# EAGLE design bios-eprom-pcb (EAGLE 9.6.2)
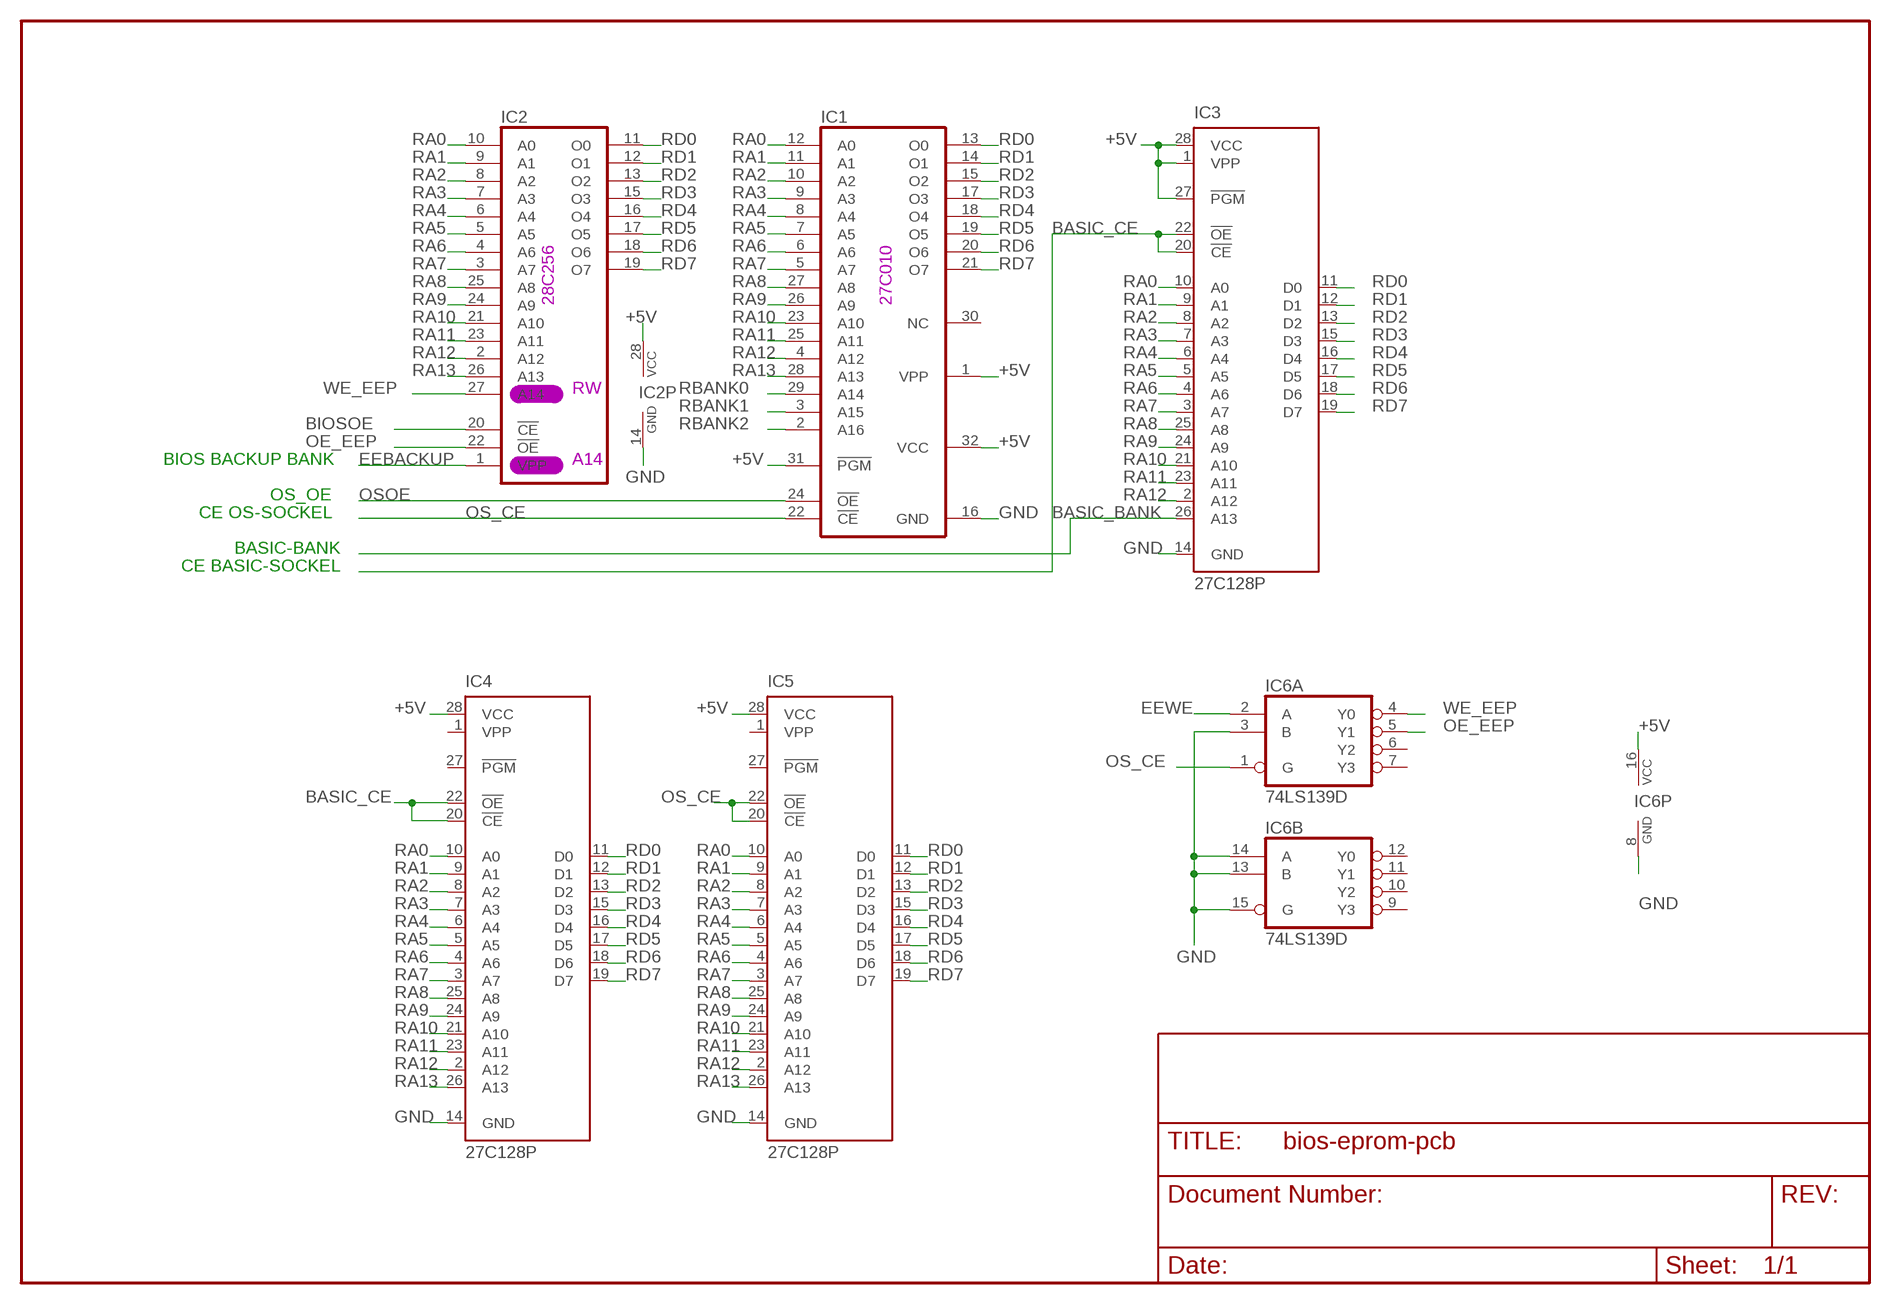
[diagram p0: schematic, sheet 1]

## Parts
IC1  27C1001A  [DIL32]
IC2  27256  [DIL28]
IC3  27C128P  [DIL28-6]
IC4  27C128P  [DIL28-6]
IC5  27C128P  [DIL28-6]
IC6  74LS139D  [SO16]

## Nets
+5V: IC1.1(VPP) IC1.31(!PGM) IC1.32(VCC) IC2.28(VCC) IC3.1(VPP) IC3.27(!PGM) IC3.28(VCC) IC4.28(VCC) IC5.28(VCC) IC6.16(P:VCC)
BASIC_BANK: IC3.26(A13)
BASIC_CE: IC3.20(!CE) IC3.22(!OE) IC4.20(!CE) IC4.22(!OE)
BIOSOE: IC2.20(!CE)
EEBACKUP: IC2.1(VPP)
EEWE: IC6.2(A:A)
GND: IC1.16(GND) IC2.14(GND) IC3.14(GND) IC4.14(GND) IC5.14(GND) IC6.3(A:B) IC6.8(P:GND) IC6.13(B:B) IC6.14(B:A) IC6.15(B:G)
OE_EEP: IC2.22(!OE) IC6.5(A:Y1)
OS_CE: IC1.22(!CE) IC5.20(!CE) IC5.22(!OE) IC6.1(A:G)
OSOE: IC1.24(!OE)
RA0: IC1.12(A0) IC2.10(A0) IC3.10(A0) IC4.10(A0) IC5.10(A0)
RA1: IC1.11(A1) IC2.9(A1) IC3.9(A1) IC4.9(A1) IC5.9(A1)
RA2: IC1.10(A2) IC2.8(A2) IC3.8(A2) IC4.8(A2) IC5.8(A2)
RA3: IC1.9(A3) IC2.7(A3) IC3.7(A3) IC4.7(A3) IC5.7(A3)
RA4: IC1.8(A4) IC2.6(A4) IC3.6(A4) IC4.6(A4) IC5.6(A4)
RA5: IC1.7(A5) IC2.5(A5) IC3.5(A5) IC4.5(A5) IC5.5(A5)
RA6: IC1.6(A6) IC2.4(A6) IC3.4(A6) IC4.4(A6) IC5.4(A6)
RA7: IC1.5(A7) IC2.3(A7) IC3.3(A7) IC4.3(A7) IC5.3(A7)
RA8: IC1.27(A8) IC2.25(A8) IC3.25(A8) IC4.25(A8) IC5.25(A8)
RA9: IC1.26(A9) IC2.24(A9) IC3.24(A9) IC4.24(A9) IC5.24(A9)
RA10: IC1.23(A10) IC2.21(A10) IC3.21(A10) IC4.21(A10) IC5.21(A10)
RA11: IC1.25(A11) IC2.23(A11) IC3.23(A11) IC4.23(A11) IC5.23(A11)
RA12: IC1.4(A12) IC2.2(A12) IC3.2(A12) IC4.2(A12) IC5.2(A12)
RA13: IC1.28(A13) IC2.26(A13) IC4.26(A13) IC5.26(A13)
RBANK0: IC1.29(A14)
RBANK1: IC1.3(A15)
RBANK2: IC1.2(A16)
RD0: IC1.13(O0) IC2.11(O0) IC3.11(D0) IC4.11(D0) IC5.11(D0)
RD1: IC1.14(O1) IC2.12(O1) IC3.12(D1) IC4.12(D1) IC5.12(D1)
RD2: IC1.15(O2) IC2.13(O2) IC3.13(D2) IC4.13(D2) IC5.13(D2)
RD3: IC1.17(O3) IC2.15(O3) IC3.15(D3) IC4.15(D3) IC5.15(D3)
RD4: IC1.18(O4) IC2.16(O4) IC3.16(D4) IC4.16(D4) IC5.16(D4)
RD5: IC1.19(O5) IC2.17(O5) IC3.17(D5) IC4.17(D5) IC5.17(D5)
RD6: IC1.20(O6) IC2.18(O6) IC3.18(D6) IC4.18(D6) IC5.18(D6)
RD7: IC1.21(O7) IC2.19(O7) IC3.19(D7) IC4.19(D7) IC5.19(D7)
WE_EEP: IC2.27(A14) IC6.4(A:Y0)
Unconnected: IC1.30(NC) IC4.1(VPP) IC4.27(!PGM) IC5.1(VPP) IC5.27(!PGM) IC6.6(A:Y2) IC6.7(A:Y3) IC6.9(B:Y3) IC6.10(B:Y2) IC6.11(B:Y1) IC6.12(B:Y0)

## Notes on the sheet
- 28C256 | 27C010
- RW
- BIOS BACKUP BANK | A14
- OS_OE
- CE OS-SOCKEL
- BASIC-BANK
- CE BASIC-SOCKEL

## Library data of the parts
IC1 = memory-nec:27C1001A: MEMORY; MPN: M27C1001-15F1; OC_FARNELL: 1661756; OC_NEWARK: 78M7615
IC2 = memory:27256: MEMORY
IC3-IC5 = microchip:27*128: CMOS EPROM 128 K (16 K x 8); OC_FARNELL: unknown; OC_NEWARK: unknown
IC6 = 74xx-eu:74*139: Dual 2-line to 4-line DECODER/DEMULTIPLEXER

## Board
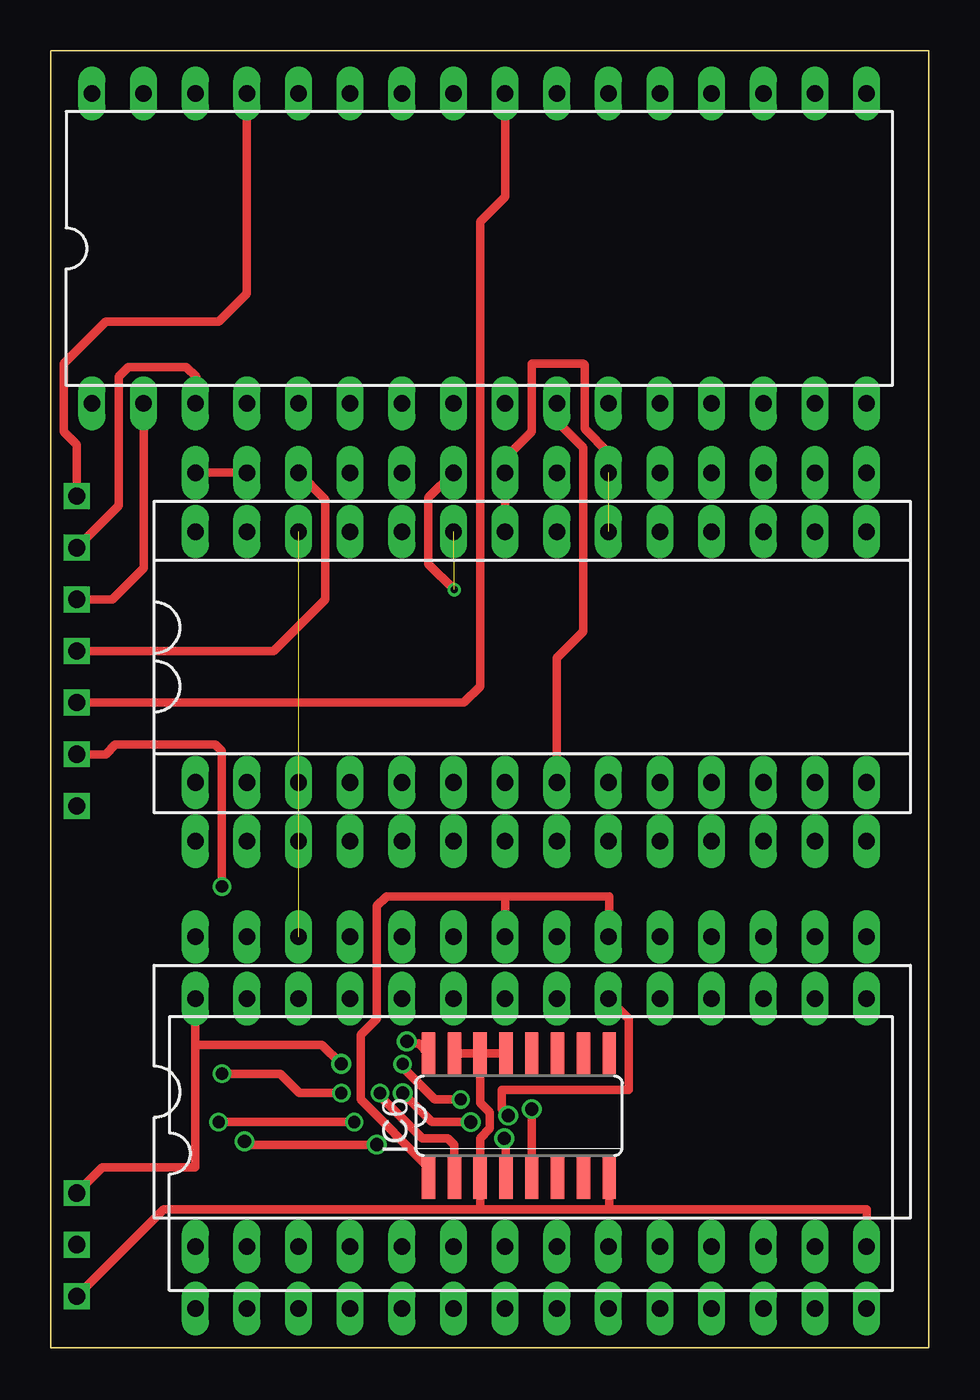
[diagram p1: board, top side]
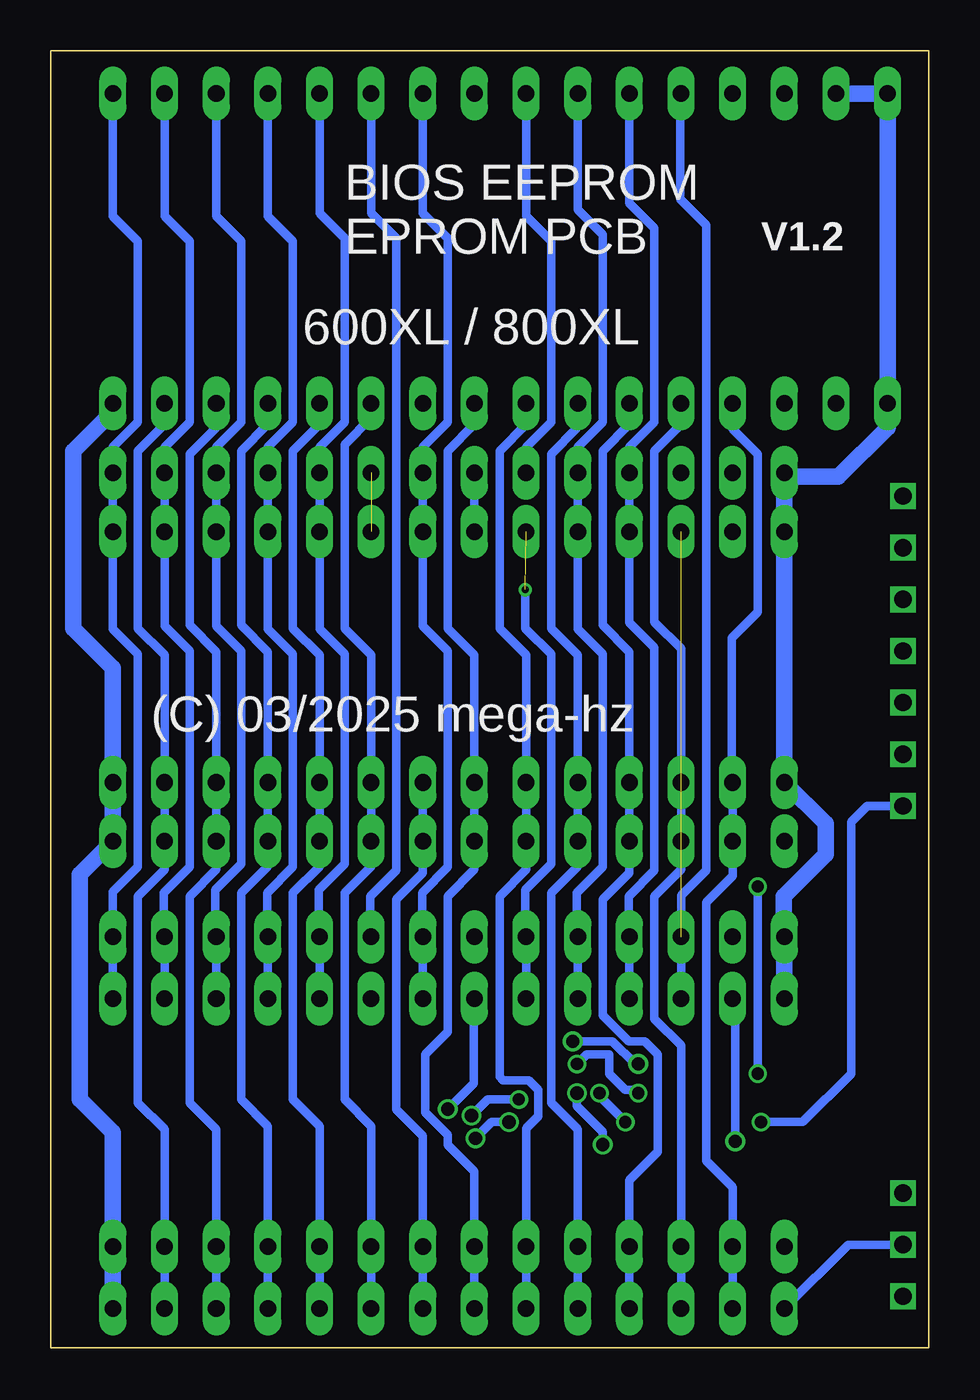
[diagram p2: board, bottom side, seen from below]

Size 43.18 x 63.82 mm. Coordinates in mm from the lower left corner, seen from the top.
Outline: 43.18,0 43.18,63.82 0,63.82 0,0 43.18,0
Copper layers (1+2*15+16): Top 0.035mm / dielectric 1.5mm / Route2 0.035mm / dielectric 0.15mm / Route15 0.035mm / dielectric 0.2mm / Bottom 0.035mm
Design rules "ITead_rule *": minimum track width 6mil, minimum drill 12mil, track to track 6mil, track to pad 6mil, pad to pad 6mil, via to via 6mil, smd to smd 0mil, copper to edge 10mil, drill to drill 10mil, minimum pad ring 10mil, minimum via ring 6mil, stop-mask expansion 2mil, vias tented up to drill 100mil, thermal gap 10mil

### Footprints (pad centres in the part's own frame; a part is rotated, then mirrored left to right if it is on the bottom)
DIL32 = drill 0.813 long: 1 -19.05,-7.62; 2 -16.51,-7.62; 3 -13.97,-7.62; 4 -11.43,-7.62; 5 -8.89,-7.62; 6 -6.35,-7.62; 7 -3.81,-7.62; 8 -1.27,-7.62; 9 1.27,-7.62; 10 3.81,-7.62; 11 6.35,-7.62; 12 8.89,-7.62; 13 11.43,-7.62; 14 13.97,-7.62; 15 16.51,-7.62; 16 19.05,-7.62; 17 19.05,7.62; 18 16.51,7.62; 19 13.97,7.62; 20 11.43,7.62; 21 8.89,7.62; 22 6.35,7.62; 23 3.81,7.62; 24 1.27,7.62; 25 -1.27,7.62; 26 -3.81,7.62; 27 -6.35,7.62; 28 -8.89,7.62; 29 -11.43,7.62; 30 -13.97,7.62; 31 -16.51,7.62; 32 -19.05,7.62
DIL28 = drill 0.813 long: 1 -16.51,-7.62; 2 -13.97,-7.62; 3 -11.43,-7.62; 4 -8.89,-7.62; 5 -6.35,-7.62; 6 -3.81,-7.62; 7 -1.27,-7.62; 8 1.27,-7.62; 9 3.81,-7.62; 10 6.35,-7.62; 11 8.89,-7.62; 12 11.43,-7.62; 13 13.97,-7.62; 14 16.51,-7.62; 15 16.51,7.62; 16 13.97,7.62; 17 11.43,7.62; 18 8.89,7.62; 19 6.35,7.62; 20 3.81,7.62; 21 1.27,7.62; 22 -1.27,7.62; 23 -3.81,7.62; 24 -6.35,7.62; 25 -8.89,7.62; 26 -11.43,7.62; 27 -13.97,7.62; 28 -16.51,7.62
DIL28-6 = drill 0.813 long: 1 -16.51,-7.62; 2 -13.97,-7.62; 3 -11.43,-7.62; 4 -8.89,-7.62; 5 -6.35,-7.62; 6 -3.81,-7.62; 7 -1.27,-7.62; 8 1.27,-7.62; 9 3.81,-7.62; 10 6.35,-7.62; 11 8.89,-7.62; 12 11.43,-7.62; 13 13.97,-7.62; 14 16.51,-7.62; 15 16.51,7.62; 16 13.97,7.62; 17 11.43,7.62; 18 8.89,7.62; 19 6.35,7.62; 20 3.81,7.62; 21 1.27,7.62; 22 -1.27,7.62; 23 -3.81,7.62; 24 -6.35,7.62; 25 -8.89,7.62; 26 -11.43,7.62; 27 -13.97,7.62; 28 -16.51,7.62
SO16 = smd 0.66 x 2.032: 1 -4.445,-3.073; 2 -3.175,-3.073; 3 -1.905,-3.073; 4 -0.635,-3.073; 5 0.635,-3.073; 6 1.905,-3.073; 7 3.175,-3.073; 8 4.445,-3.073; 9 4.445,3.073; 10 3.175,3.073; 11 1.905,3.073; 12 0.635,3.073; 13 -0.635,3.073; 14 -1.905,3.073; 15 -3.175,3.073; 16 -4.445,3.073

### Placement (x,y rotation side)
IC1  21.07,54.09 0 top
IC2  23.61,9.56 0 top
IC3  23.61,35.44 0 top
IC4  23.61,32.54 0 top
IC5  23.61,12.6 0 top
IC6  23.02,11.43 0 top

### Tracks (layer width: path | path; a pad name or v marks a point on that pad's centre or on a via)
+5V  (via drill 0.65, 0.85)
  Top 0.406: v1.27,7.62 2.54,8.89 7.1,8.89 7.1,14.92 | 7.1,14.92 IC2.28 | IC6.16 18.1,14.98 17.51,14.98 v17.51,15.08 | v14.29,13.97 13.34,14.92 7.1,14.92 | IC3.28 IC3.27
  Bottom 0.406: v17.51,15.08 15.56,15.08 14.45,13.97 v14.29,13.97
  Bottom 0.813: IC1.31 IC1.32 IC1.1 2.02,45.28 4.45,42.86 6.91,42.86 IC3.28 IC4.28 IC3.1 5.08,25.8 5.08,24.29 7.14,22.23 7.14,20.26 IC5.28 IC2.28
BASIC_BANK  (via drill 0.85)
  Top 0.406: v1.27,34.29 10.95,34.29 13.49,36.83 13.49,41.75 IC3.26
BASIC_CE  (1 unrouted)
  Top 0.406: IC4.22 22.34,43.77 23.65,45.09 23.65,48.42 26.19,48.42 26.25,48.36 26.25,45.23 27.42,44.06 IC3.20
  Bottom 0.406: IC4.22 IC3.22
BIOSOE  (via drill 0.6, 0.65, 0.85)
  Top 0.406: v20.16,12.22 18.89,12.22 17.3,13.81 v17.3,13.97 | v14.29,12.54 12.22,12.54 11.27,13.49 v8.41,13.49 | v8.41,22.7 8.41,29.37 8.1,29.69 3.17,29.69 2.7,29.21 v1.27,29.21 | v22.49,11.43 22.18,11.75 22.18,12.7 28.42,12.7 28.42,16.19 IC2.20
  Bottom 0.406: v20.16,12.22 21.7,12.22 v22.49,11.43 | v17.3,13.97 16.83,14.45 15.72,14.45 15.72,13.49 14.92,12.7 14.45,12.7 v14.29,12.54 | v8.41,13.49 v8.41,22.7
EEBACKUP  (via drill 0.85)
  Bottom 0.406: v1.27,5.08 3.97,5.08 IC2.1
EEWE  (via drill 0.6, 0.85)
  Top 0.406: IC6.2 19.84,10 19.53,10.32 18.26,10.32 16.19,12.38 v16.19,12.54 | v14.92,11.11 v8.26,11.11
  Bottom 0.406: v16.19,12.54 16.19,12.38 v14.92,11.11 | v8.26,11.11 6.19,11.11 3.81,13.49 3.81,25.88 3.02,26.67 v1.27,26.67
GND  (via drill 0.85)
  Top 0.406: v1.27,2.54 5.56,6.83 21.11,6.83 | IC5.14 40.12,6.83 27.46,6.83 | 21.11,6.83 27.46,6.83 | IC6.8 27.46,6.83 | 21.11,6.83 IC6.3 21.11,10.32 21.59,10.79 21.59,11.59 21.11,12.06 IC6.14 | IC6.15 IC6.14 | IC6.14 IC6.13
  Bottom 0.813: IC1.16 40.12,46.08 42.07,44.13 42.07,35.4 40.12,33.46 IC3.14 IC4.14 41.75,23.3 41.75,12.22 40.12,10.6 IC5.14 IC2.14
OE_EEP  (via drill 0.65)
  Top 0.406: v23.65,11.75 IC6.5
  Bottom 0.406: v23.65,11.75 22.38,13.02 22.38,17.14 IC2.22
OS_CE
  Top 0.406: IC6.1 18.57,8.89 15.24,12.22 15.24,15.4 16.03,16.19 16.03,21.75 16.51,22.23 22.38,22.23 | IC5.22 22.34,22.18 22.38,22.23 | 22.38,22.23 27.46,22.23 27.46,20.26 IC5.20
  Bottom 0.406: IC1.22 27.42,55.84 26.19,54.61 26.19,23.5 27.46,22.23 27.46,20.26 IC5.20
OSOE  (via drill 0.85)
  Top 0.406: IC1.24 22.34,56.63 21.11,55.4 21.11,32.54 20.32,31.75 v1.27,31.75
RA0
  Bottom 0.406: IC2.10 IC5.10 29.96,10.91 31.27,12.22 31.27,22.38 29.96,23.69 IC4.10 IC3.10 29.96,34.09 31.27,35.4 31.27,44.13 29.96,45.44 IC1.12
RA1
  Bottom 0.406: IC1.11 27.42,45.76 28.73,44.45 28.73,35.4 27.42,34.09 IC3.9 IC4.9 27.42,23.69 28.73,22.38 28.73,12.22 27.42,10.91 IC5.9 IC2.9
RA2
  Top 0.406: IC3.8 24.88,33.93 26.19,35.24 26.19,44.29 24.88,45.6 IC1.10
  Bottom 0.406: IC2.8 IC5.8 24.88,10.44 26.19,11.75 26.19,22.07 24.88,23.38 IC4.8 IC3.8
RA3
  Bottom 0.406: IC1.9 22.34,45.44 23.65,44.13 23.65,35.4 22.34,34.09 IC3.7 IC4.7 22.34,23.54 23.65,22.23 23.65,15.56 24.77,14.45 24.77,11.59 23.65,10.48 23.65,10 22.34,8.69 IC5.7 IC2.7
RA4
  Bottom 0.406: IC2.6 IC5.6 19.8,10.79 19.21,11.39 19.21,12.7 19.68,13.18 20.95,13.18 21.11,13.34 21.11,22.23 19.8,23.54 IC4.6 IC3.6 19.8,34.09 21.11,35.4 21.11,44.13 19.8,45.44 IC1.8
RA5
  Bottom 0.406: IC1.7 17.3,46.44 17.3,45.24 18.57,43.97 18.57,35.4 17.26,34.09 IC3.5 IC4.5 17.26,23.69 18.57,22.38 18.57,12.06 17.26,10.76 IC5.5 IC2.5
RA6
  Bottom 0.406: IC2.4 IC5.4 14.72,8.26 13.34,9.64 13.34,14.45 13.97,15.08 14.76,15.08 16.03,16.35 16.03,22.07 14.72,23.38 IC4.4 IC3.4 14.72,34.25 16.03,35.56 16.03,44.13 14.72,45.44 IC1.6
RA7
  Bottom 0.406: IC1.5 12.18,45.44 13.49,44.13 13.49,35.72 12.18,34.41 IC3.3 IC4.3 12.18,23.54 13.49,22.23 13.49,16.19 12.18,14.88 IC5.3 IC2.3
RA8
  Bottom 0.406: IC1.27 14.72,56.32 13.49,55.09 13.49,45.56 14.72,44.33 IC3.25 IC4.25 14.72,35.68 13.49,34.45 13.49,23.5 14.76,22.23 14.76,20.26 IC5.25 IC2.25
RA9
  Bottom 0.406: IC1.26 17.26,56 16.03,54.77 16.03,45.56 17.26,44.33 IC3.24 IC4.24 17.26,35.36 16.03,34.13 16.03,23.65 17.3,22.38 17.3,20.26 IC5.24 IC2.24
RA10
  Bottom 0.406: IC1.23 24.88,55.84 23.65,54.61 23.65,45.56 24.88,44.33 IC3.21 IC4.21 24.88,35.52 23.65,34.29 23.65,23.65 24.92,22.38 24.92,20.26 IC5.21 IC2.21
RA11  (via drill 0.35)  (1 unrouted)
  Top 0.406: v19.84,37.31 18.57,38.58 18.57,41.83 IC3.23
  Bottom 0.406: IC1.25 19.8,55.68 18.57,54.45 18.57,45.56 19.8,44.33 IC3.23 | IC2.23 IC5.23 19.84,20.26 19.84,22.54 18.57,23.81 18.57,34.13 19.84,35.4 v19.84,37.31
RA12
  Bottom 0.406: IC1.4 9.64,45.2 8.41,43.97 8.41,36.2 9.68,34.92 9.68,27.86 IC3.2 IC4.2 9.64,23.22 10.95,21.91 10.95,9.21 9.64,7.9 IC5.2 IC2.2
RA13  (1 unrouted)
  Bottom 0.406: IC2.26 IC5.26 12.18,22.27 10.95,23.5 10.95,35.88 10.95,55.24 12.22,56.52 12.22,61.67 IC1.28
RBANK0  (via drill 0.85)
  Top 0.406: v1.27,41.91 1.27,44.45 0.64,45.09 0.64,48.42 2.7,50.48 8.26,50.48 9.64,51.87 IC1.29
RBANK1  (via drill 0.85)
  Top 0.406: v1.27,39.37 3.33,41.43 3.33,47.78 3.81,48.26 6.67,48.26 7.14,47.78 7.14,46.51 IC1.3
RBANK2  (via drill 0.85)
  Top 0.406: v1.27,36.83 3.02,36.83 4.56,38.38 IC1.2
RD0
  Bottom 0.406: IC1.13 32.5,45.44 33.81,44.13 33.81,35.56 32.5,34.25 IC3.11 IC4.11 32.5,23.69 33.81,22.38 33.81,12.22 32.5,10.91 IC5.11 IC2.11
RD1
  Bottom 0.406: IC2.12 IC5.12 35.04,10.76 36.35,12.06 36.35,22.23 35.04,23.54 IC4.12 IC3.12 35.04,34.25 36.35,35.56 36.35,43.97 35.04,45.28 IC1.14
RD2
  Bottom 0.406: IC1.15 37.58,45.44 38.89,44.13 38.89,35.4 37.58,34.09 IC3.13 IC4.13 37.58,23.54 38.89,22.23 38.89,12.06 37.58,10.76 IC5.13 IC2.13
RD3
  Bottom 0.406: IC1.17 40.12,55.68 38.89,54.45 38.89,45.56 40.12,44.33 IC3.15 IC4.15 40.12,35.36 38.89,34.13 38.89,23.65 40.12,22.42 IC5.15 IC2.15
RD4
  Bottom 0.406: IC1.18 37.58,55.68 36.35,54.45 36.35,45.56 37.58,44.33 IC3.16 IC4.16 37.58,35.52 36.35,34.29 36.35,23.65 37.62,22.38 37.62,20.26 IC5.16 IC2.16
RD5
  Bottom 0.406: IC1.19 35.04,55.68 33.81,54.45 33.81,45.56 35.04,44.33 IC3.17 IC4.17 35.04,35.52 33.81,34.29 33.81,23.81 35.08,22.54 35.08,20.26 IC5.17 IC2.17
RD6
  Bottom 0.406: IC1.20 32.5,55.68 31.27,54.45 31.27,45.56 32.5,44.33 IC3.18 IC4.18 32.5,35.36 31.27,34.13 31.27,23.65 32.54,22.38 32.54,20.26 IC5.18 IC2.18
RD7
  Bottom 0.406: IC1.21 29.96,55.84 28.73,54.61 28.73,45.56 29.96,44.33 IC3.19 IC4.19 29.96,35.36 28.73,34.13 28.73,23.81 30,22.54 30,20.26 IC5.19 IC2.19
WE_EEP  (via drill 0.65)
  Top 0.406: v20.65,11.11 18.73,11.11 v17.3,12.54 | v16.03,10 9.68,10 v9.53,10.16 | v22.3,10.32 22.38,10.23 IC6.4
  Bottom 0.406: v22.3,10.32 21.5,11.11 v20.65,11.11 | v17.3,12.54 17.3,11.91 16.03,10.64 v16.03,10 | v9.53,10.16 9.53,17.07 IC2.27

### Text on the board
bPlace: V1.2 | BIOS EEPROM / EPROM PCB | 600XL / 800XL | (C) 03/2025 mega-hz
Gehäuse: 27C010 | 8xOS | 1 | B0 | 2 | B1 | 3 | B2 | 27C128 | 4 | B3 | 5 | 2xBASIC | XL | 6 | OS | BIOS | 7 | EE | WE | (C)2025 mega-hz | 28C256 | 74LS139 | ATARI BIOS | ATARI BIOS | ATARI BIOS | BIOS | EEPROM | BACKUP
